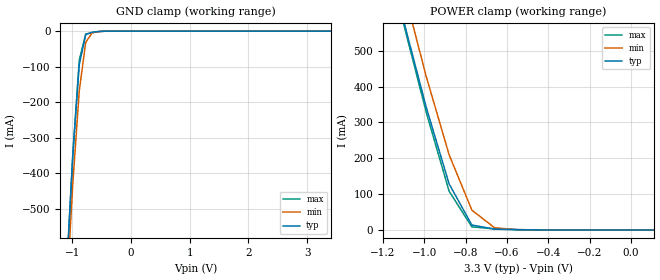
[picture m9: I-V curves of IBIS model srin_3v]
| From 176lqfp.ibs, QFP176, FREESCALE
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[Model] srin_3v
|   Model srin_3v
Model_type Input
Polarity   Non-Inverting
Enable   Active-High
Vinl =   1.1500V
Vinh =   2.1500V
C_comp   4.7071pF   4.5259pF   4.9715pF
[Temperature Range]   25.0000   0.1500k   -40.0000
[Voltage Range]   3.3000V   2.9700V   3.6300V
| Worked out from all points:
|   GND clamp passes 1 mA (typ) near -0.56 V on its own axis
|   POWER clamp passes 1 mA (typ) near -0.57 V on its own axis
[GND_clamp]
|Voltage   I(typ)   I(min)   I(max)
-3.63V    -10.2A     -10.16A    -10.28A
-1.1V     -683.5mA   -753.4mA   -695.2mA
-990mV    -349.5mA   -429.8mA   -348.6mA
-880mV    -94.6mA    -168.5mA   -81.78mA
-770mV    -9.279mA   -31.37mA   -8.242mA
-660mV    -2.916mA   -4.583mA   -4.405mA
-440mV    -65.66uA   -239.8uA   -36.5uA
3.41V     626.5pA    220.2uA    6.002pA
[POWER_clamp]
|Voltage   I(typ)   I(min)   I(max)
-3.63V    7.308A     7.439A     7.307A
-1.1V     583.2mA    670.8mA    574.6mA
-990mV    341mA      426.7mA    326.9mA
-880mV    128.5mA    209.9mA    108.2mA
-770mV    13.88mA    55.46mA    8.676mA
-660mV    2.265mA    6.121mA    3.037mA
-550mV    681.9uA    981.3uA    900.8uA
110mV     37.89pA    5.502nA    6.134pA
